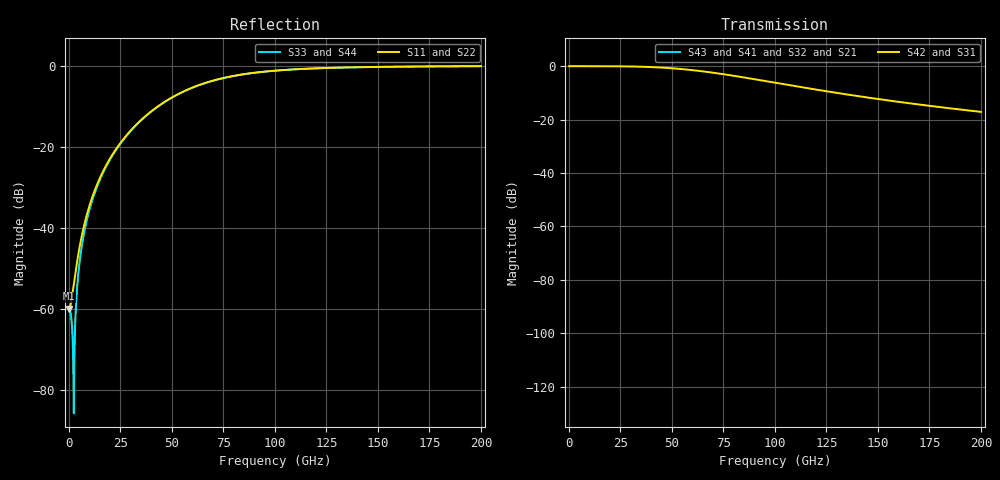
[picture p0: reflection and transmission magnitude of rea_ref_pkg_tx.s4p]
! Created with skrf 1.10.0 (http://scikit-rf.org).
# Hz S RI R 50.0
!freq ReS11 ImS11 ReS12 ImS12 ReS13 ImS13
! ReS14 ImS14
! ReS21 ImS21 ReS22 ImS22 ReS23 ImS23
! ReS24 ImS24
! ReS31 ImS31 ReS32 ImS32 ReS33 ImS33
! ReS34 ImS34
! ReS41 ImS41 ReS42 ImS42 ReS43 ImS43
! ReS44 ImS44
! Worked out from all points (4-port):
!   2000 points, 100 MHz to 200 GHz, reference 50 ohm
!   strongest paths, dB at 100 MHz, 50.1 GHz, 100.1 GHz, 150.1 GHz, 200 GHz:
!     S42: 0.0, -0.8, -6.2, -12.3, -17.1
!     S31: 0.0, -0.8, -6.2, -12.3, -17.1
!     S43: -, -, -, -, -
!     S41: -, -, -, -, -
!     S32: -, -, -, -, -
!     S21: -, -, -, -, -
!   lowest |S11| = -60.0 dB at 100 MHz (marker M1), VSWR 1.00, Z = 50.1 - j0.000378 ohm
!   |S11| at or under -10 dB: start of sweep to 43.27 GHz
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1e8  0.001 -3.77e-06  0 0  0.999 -0.00188  0 0
     0 0  0.001 -3.77e-06  0 0  0.999 -0.00188
     0.999 -0.00188  0 0  0.000997 3.34e-09  0 0
     0 0  0.999 -0.00188  0 0  0.000997 3.34e-09
2.4e9  0.00202 -0.000137  0 0  0.998 -0.0452  0 0
       0 0  0.00202 -0.000137  0 0  0.998 -0.0452
       0.998 -0.0452  0 0  -2.12e-05 4.62e-05  0 0
       0 0  0.998 -0.0452  0 0  -2.12e-05 4.62e-05
6.8e9  0.00911 -0.00131  0 0  0.9907 -0.128  0 0
       0 0  0.00911 -0.00131  0 0  0.9907 -0.128
       0.9907 -0.128  0 0  -0.00713 0.00105  0 0
       0 0  0.9907 -0.128  0 0  -0.00713 0.00105
1.66e10  0.0472 -0.0159  0 0  0.9478 -0.3118  0 0
         0 0  0.0472 -0.0159  0 0  0.9478 -0.3118
         0.9478 -0.3118  0 0  -0.0454 0.0152  0 0
         0 0  0.9478 -0.3118  0 0  -0.0454 0.0152
4.89e10  0.2066 -0.3325  0 0  0.4869 -0.7797  0 0
         0 0  0.2066 -0.3325  0 0  0.4869 -0.7797
         0.4869 -0.7797  0 0  -0.2056 0.3309  0 0
         0 0  0.4869 -0.7797  0 0  -0.2056 0.3309
9.6e10  -0.2837 -0.8048  0 0  -0.1726 -0.4914  0 0
        0 0  -0.2837 -0.8048  0 0  -0.1726 -0.4914
        -0.1726 -0.4914  0 0  0.2833 0.8038  0 0
        0 0  -0.1726 -0.4914  0 0  0.2833 0.8038
2e11  -0.8426 -0.5202  0 0  -0.1185 -0.0733  0 0
      0 0  -0.8426 -0.5202  0 0  -0.1185 -0.0733
      -0.1185 -0.0733  0 0  0.8423 0.5201  0 0
      0 0  -0.1185 -0.0733  0 0  0.8423 0.5201
